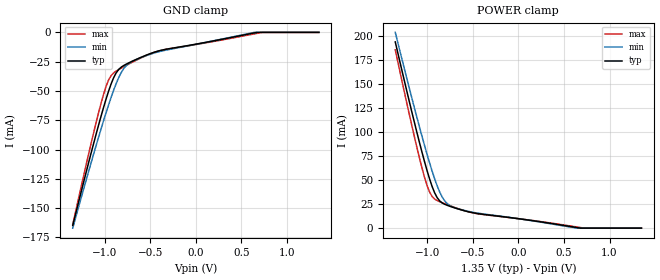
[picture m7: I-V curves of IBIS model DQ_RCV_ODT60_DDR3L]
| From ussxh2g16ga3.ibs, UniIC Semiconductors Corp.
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|   Model DQ_RCV_ODT60_DDR3L
[Model] DQ_RCV_ODT60_DDR3L
Model_type Input
Vinl =  0.540V
Vinh =  0.810V
C_comp   0.966pF   0.965pF   0.967pF
[Model Spec]
Vinh   0.810V   0.776V   0.860V
Vinl   0.540V   0.506V   0.590V
[Temperature Range]   25.000   95.000   -40.000
[Voltage Range]   1.350V   1.283V   1.450V
[GND_clamp]
|Voltage   I(typ)   I(min)   I(max)
-1.35V    -164.8mA   -167.1mA   -163.9mA
-1.154V   -104.6mA   -112.7mA   -96.47mA
-1.014V   -64.57mA   -75.87mA   -53.34mA
-958mV    -50.39mA   -62.12mA   -40.82mA
-930mV    -44.15mA   -55.6mA    -36.98mA
-874mV    -34.58mA   -43.7mA    -33.06mA
-818mV    -29.66mA   -34.23mA   -30.52mA
-762mV    -27.06mA   -28.26mA   -28.15mA
-706mV    -24.96mA   -25.14mA   -25.85mA
-342mV    -14.65mA   -15.36mA   -14.71mA
638mV     -505uA     -51.4uA    -1.331mA
1.35V     0A         0A         0A
[POWER_clamp]
|Voltage   I(typ)   I(min)   I(max)
-1.35V    193.8mA    203.7mA    185.5mA
-1.114V   100.1mA    115.8mA    84.5mA
-1.058V   79.44mA    96.01mA    63mA
-1.002V   60.15mA    77.1mA     44.58mA
-946mV    43.43mA    59.47mA    32.94mA
-890mV    31.65mA    43.97mA    28.68mA
-834mV    26.13mA    32.14mA    26.39mA
-778mV    23.66mA    25.3mA     24.33mA
-694mV    20.96mA    21.14mA    21.39mA
-470mV    15.53mA    16mA       15.32mA
622mV     886.5uA    316.9uA    1.502mA
1.35V     0A         0A         0A
